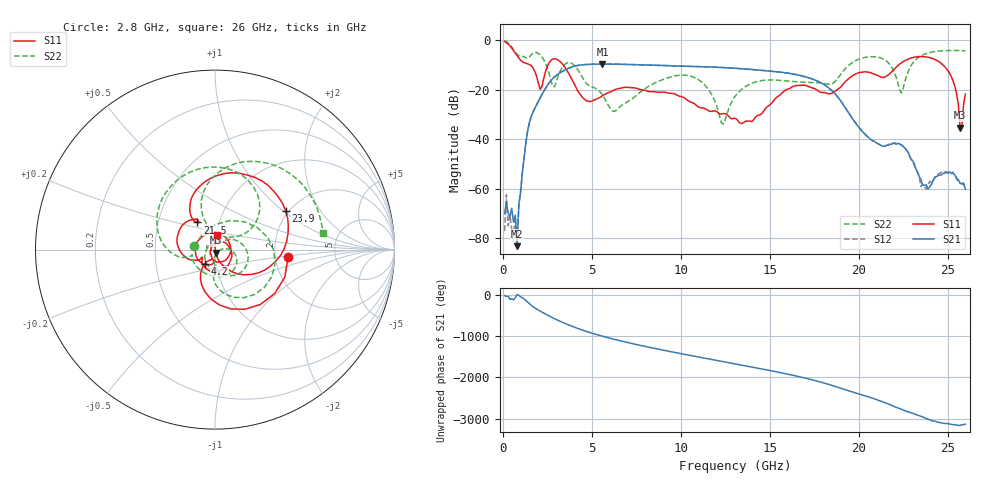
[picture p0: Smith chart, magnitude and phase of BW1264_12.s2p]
!Keysight Technologies,N5245B,MY57181159,A.13.60.06
!Date: Friday, December 18, 2020 23:52:32
!Correction: S11(Full 2 Port(1,2))
!S21(Full 2 Port(1,2))
!S12(Full 2 Port(1,2))
!S22(Full 2 Port(1,2))
!S2P File: Measurements: S11, S21, S12, S22:
# Hz S  dB  R 50
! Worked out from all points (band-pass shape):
!   260 points, 100 MHz to 26 GHz, reference 50 ohm
!   highest |S21| = -9.73 dB at 5.6 GHz (marker M1); lowest = -83.2 dB at 800 MHz (marker M2)
!   |S21| within 3 dB of the highest: 3.334 GHz to 15.3 GHz (11.97 GHz wide, 128 % of centre)
!   lowest |S11| = -35.4 dB at 25.7 GHz (marker M3), VSWR 1.03, Z = 50.4 - j1.67 ohm
!   |S11| at or under -10 dB: 1.519 GHz to 2.547 GHz (1.028 GHz wide, 50.5 % of centre); 3.38 GHz to 22.26 GHz (18.88 GHz wide, 147 % of centre); 24.73 GHz to end of sweep
!   |S22| runs from -33.9 to -0.2 dB; largest |S21 - S12| = 0.0005
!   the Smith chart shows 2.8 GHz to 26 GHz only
!   S11 on the Smith chart (normalised r, x): 2.8 GHz: 2.36, -0.22; 4.2 GHz: 0.88, -0.14; 21.5 GHz: 0.79, +0.25; 23.9 GHz: 1.94, +1.04; 26 GHz: 1.01, +0.16
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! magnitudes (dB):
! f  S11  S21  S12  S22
! 100 MHz  -0.6  -70.0  -77.0  -0.2
! 200 MHz  -1.1  -65.5  -62.4  -0.6
! 300 MHz  -1.7  -69.8  -75.0  -1.2
! 800 MHz  -6.3  -83.2  -81.4  -5.8
! 1.5 GHz  -9.9  -33.2  -33.1  -6.8
! 2.1 GHz  -19.9  -23.3  -23.3  -6.0
! 2.8 GHz  -7.8  -15.6  -15.6  -18.6
! 4.2 GHz  -20.4  -10.3  -10.3  -11.9
! 4.5 GHz  -23.3  -10.0  -10.0  -15.5
! 5.6 GHz  -22.5  -9.7  -9.7  -22.1
! 8.8 GHz  -21.1  -10.2  -10.2  -16.5
! 11 GHz  -27.0  -10.8  -10.8  -16.0
! 12.4 GHz  -29.7  -11.1  -11.1  -33.9
! 13.1 GHz  -31.7  -11.4  -11.4  -22.3
! 17.4 GHz  -19.3  -15.8  -15.7  -17.1
! 21.5 GHz  -14.9  -42.7  -42.7  -8.2
! 21.7 GHz  -13.9  -42.4  -42.0  -9.5
! 22.4 GHz  -9.3  -42.4  -42.3  -21.4
! 23.9 GHz  -7.0  -60.1  -58.6  -5.3
! 25.2 GHz  -14.7  -53.7  -53.9  -4.3
! 25.7 GHz  -35.4  -57.7  -57.8  -4.3
! 26 GHz  -21.8  -60.2  -59.4  -4.3
